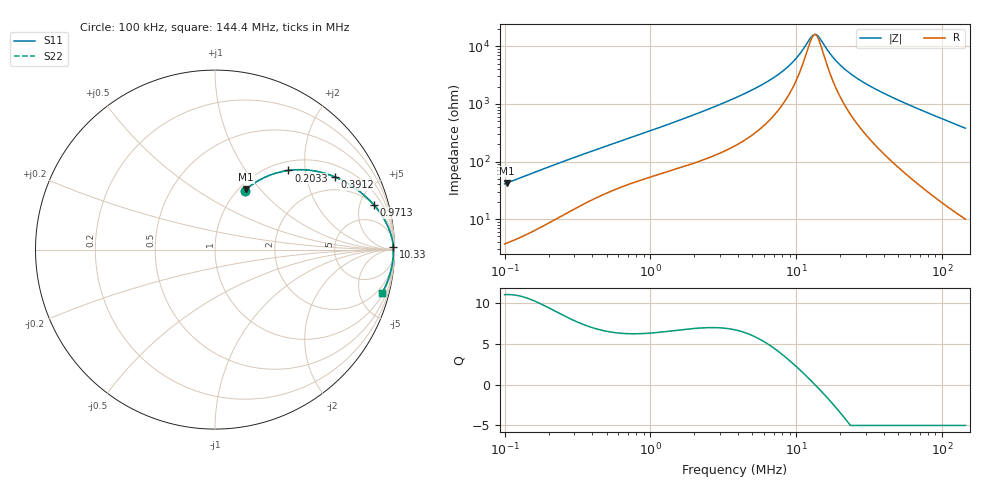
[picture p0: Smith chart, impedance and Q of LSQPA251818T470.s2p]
! LSQPA251818T470  S-PARAMETER MODEL  ( General Type )
! Model Generated by TAIYO YUDEN Corporation (http://www.ty-top.com)
! Version 3.0
! TAIYO YUDEN Control No. 160907NF25SB-FAC
! Copyright(c) 2007 TAIYO YUDEN CO.,LTD. All Rights Reserved.
! Product Description (link to TY-COMPAS)
! https://ds.yuden.co.jp/TYCOMPAS/or/detail?pn=LSQPA251818T470K&u=M
! Products Name : Inductors
! Characteristics :
!  Inductance : 47 uH , SRF(min) : 12 MHz , DC Resistance(max) : 2.47 Ohm
!  Rated Current : Saturation :240 mA , Temp Rise : 290 mA (40 degC)
!  Case Size : 2.5 x 1.8 / 0.098 x 0.071 [mm/inch] , Thickness : 1.8 / 0.071 [mm/inch]
!  (Conditions: Temperature = 25 degC , DC Bias Current/Voltage = 0A / 0V)
! External Node Assignments :
!  1  o---GGG---o  2
! GND o---------o GND
! Frequency Range : 0.1MHz  -  144.390904MHz  [ 402 STEP ]
# MHz S RI R 50
! Freq[MHz].  S11 Real  S11 Imag  S21 Real  S21 Imag  S12 Real  S12 Imag  S22 Real  S22 Imag
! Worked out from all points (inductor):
!   401 points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, 100 kHz to 144.4 MHz, reference 50 ohm
!   read as one part in series: L = 64.6 uH near 103.7 kHz
!   highest Q = 11 at 103.7 kHz (marker M1), where L = 64.8 uH
!   self-resonance near 13.33 MHz
!   S11 on the Smith chart (normalised r, x): 100 kHz: 1.07, +0.82; 203.3 kHz: 1.17, +1.62; 391.2 kHz: 1.42, +2.96; 971.3 kHz: 2.05, +6.59; 10.33 MHz: open; 144.4 MHz: 1.20, -7.57
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0.1  0.1648 0.3283  0.8352 -0.3283  0.8352 -0.3283  0.1648 0.3283
0.103705  0.1738 0.3362  0.8262 -0.3362  0.8262 -0.3362  0.1738 0.3362
0.203262  0.4091 0.441  0.5909 -0.441  0.5909 -0.441  0.4091 0.441
0.338238  0.6173 0.4233  0.3827 -0.4233  0.3827 -0.4233  0.6173 0.4233
0.391213  0.669 0.4046  0.331 -0.4046  0.331 -0.4046  0.669 0.4046
0.605322  0.794 0.3327  0.206 -0.3327  0.206 -0.3327  0.794 0.3327
0.971306  0.8844 0.2499  0.1156 -0.2499  0.1156 -0.2499  0.8844 0.2499
1.144052  0.9068 0.2227  0.0932 -0.2227  0.0932 -0.2227  0.9068 0.2227
2.201935  0.9627 0.1304  0.0373 -0.1304  0.0373 -0.1304  0.9627 0.1304
3.869624  0.983 0.0743  0.017 -0.0743  0.017 -0.0743  0.983 0.0743
7.0523  0.9913 0.0331  0.00866 -0.0331  0.00866 -0.0331  0.9913 0.0331
8.772371  0.9927 0.0212  0.00734 -0.0212  0.00734 -0.0212  0.9927 0.0212
10.33253  0.9933 0.0128  0.00671 -0.0128  0.00671 -0.0128  0.9933 0.0128
12.85266  0.9938 0.00206  0.00622 -0.00206  0.00622 -0.00206  0.9938 0.00206
13.32878  0.9938 0.00029  0.00618 -0.00029  0.00618 -0.00029  0.9938 0.00029
14.07625  0.9939 -0.00237  0.00613 0.00237  0.00613 0.00237  0.9939 -0.00237
18.15812  0.9938 -0.015  0.00615 0.015  0.00615 0.015  0.9938 -0.015
23.00149  0.9934 -0.0276  0.00659 0.0276  0.00659 0.0276  0.9934 -0.0276
30.21613  0.9923 -0.0441  0.00773 0.0441  0.00773 0.0441  0.9923 -0.0441
43.47261  0.9891 -0.0713  0.0109 0.0713  0.0109 0.0713  0.9891 -0.0713
80.682  0.9738 -0.14  0.0262 0.14  0.0262 0.14  0.9738 -0.14
144.3909  0.9292 -0.2436  0.0708 0.2436  0.0708 0.2436  0.9292 -0.2436
